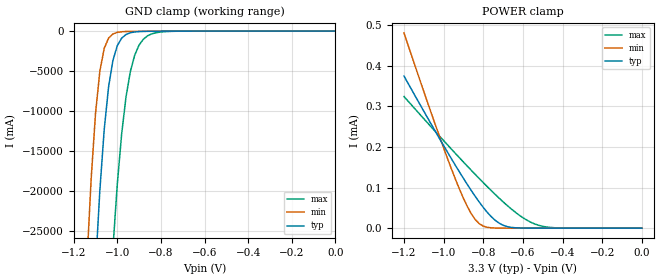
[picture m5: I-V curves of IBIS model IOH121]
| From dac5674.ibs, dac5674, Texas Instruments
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[Model]   IOH121
Model_type   Input
Polarity   Non-Inverting
| signals   Y
Vinl = 0.8V
Vinh = 2.0V
|   typ   min   max
C_comp   1.8732p   1.8084p   2.1271p
|   typ   min   max
[Temperature Range]   25   -40.0   125
|   typ   min   max
[Voltage Range]   3.30V   3.00V   3.60V
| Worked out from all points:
|   GND clamp passes 1 mA (typ) near -0.59 V on its own axis
[GND_clamp]
|   Voltage   I(typ)   I(min)   I(max)
-1.2V     -98.78A    -71.42A    -148.8A
-1.14V    -54.21A    -29.33A    -101.8A
-1.1V     -29.69A    -10.34A    -73.18A
-1.08V    -19.94A    -5.009A    -60A
-1.06V    -12.32A    -2.162A    -47.8A
-1.04V    -6.982A    -879.7mA   -36.79A
-1.02V    -3.664A    -360.7mA   -27.18A
-980mV    -883.6mA   -82.98mA   -12.87A
-960mV    -427.4mA   -52.44mA   -8.231A
-920mV    -109.8mA   -32.58mA   -3A
-880mV    -38.47mA   -25.05mA   -1.002A
0V        -6.6pA     -7.2pA     -9.285pA
[POWER_clamp]
|   Voltage   I(typ)   I(min)   I(max)
-1.2V     374.2uA    480.4uA    323.8uA
-1.04V    236.5uA    251.8uA    236.8uA
-940mV    154uA      119.8uA    183.5uA
-880mV    107.1uA    52.79uA    152.3uA
-840mV    77.73uA    20.85uA    131.9uA
-820mV    63.94uA    10.91uA    121.8uA
-760mV    28.38uA    817.7nA    92.48uA
-700mV    7.217uA    43.91nA    64.78uA
-600mV    217.9nA    452.1pA    25.71uA
-520mV    10.24nA    137.7pA    6.943uA
-420mV    349.5pA    127.9pA    575.2nA
0V        110.6pA    113.7pA    2.598nA
